//{{V2}}
FUNCTION_BLOCK FB32
TITLE=Get Homing Parameter
//*****************************************************************************
//* maxon motor ag
//* R&D
//* all rights reserved
//*****************************************************************************
//* Summary:  Read all homing parameters
//*
//* Remarks:
//*
//* Created under: STEP7 REV5.2+SP1
//*****************************************************************************
//* History:
//* 19.05.2004 | INA   first release
//*
//*
//*****************************************************************************
//


AUTHOR:INA
FAMILY:HomingMo
NAME:GetHoPa
VERSION:00.01


VAR_INPUT
       Read:BOOL //A rising edge start the command
       NodeID:BYTE //Adress of the maxon device
END_VAR

VAR_OUTPUT
       Done:BOOL //Data valid flag is TRUE if data were available
       Err:BOOL //Error flag is TRUE if an Error has occured, see ErrNo for more details
       ErrNo:DINT //Contains detailed error information
       HomingAcceleration:DWORD //Acceleration for Homing Profile
       SpeedSwitch:DWORD //Speed during search for switch
       SpeedIndex:DWORD //Speed during search for index signal
       HomeOffset:DINT //Home Offset after Homing
       CurrentThreshold:WORD //Current Threshold for Homing Method -3 and -4
       HomePosition:DINT //Home position value
END_VAR

VAR_IN_OUT
END_VAR

VAR
       xEdgeMerker:BOOL //Edge Merker
       xEdgeFlag:BOOL //Edge Flag
       xStep:INT
END_VAR

VAR_TEMP
END_VAR
BEGIN

NETWORK
TITLE= Activate the service function
//{{a}}
//

// SDO Read "Get Homing Parameter"

       U    #Read
       FP   #xEdgeFlag                   // recognize a positiv edge of the Read signal
       =    #xEdgeMerker                 // and set the xEdgeMerker for one cycle to true

       L    #xStep
       L    0
       ==I
       U    #xEdgeMerker
       SPB  nstp                         // iStep = 1 -> fnc1

       L    #xStep                       // jump list
       SPL  List
       SPA  rdef
       SPA  fnc1
       SPA  fncE
List  :SPA  rdef

rdef  :NOP  0
       R    #Done                        // reset Done
       R    #Err                         // reset Error
       L    0
       T    #xStep                       // iStep = 0
       SPA  end

fnc1  :NOP  0
       CALL FC1
         NodeID:=#NodeID
         Index:=DW#16#00006099
         SubIndex:=DW#16#00000002
         RET_VAL:=#Done
         Err:=#Err
         ErrNo:=#ErrNo

       L    DB219.DBD10
       T    #SpeedIndex

       L    1
       U    #Err
       SPB  fncE

       NOP  0
       CALL FC1
         NodeID:=#NodeID
         Index:=DW#16#0000609A
         SubIndex:=DW#16#00000000
         RET_VAL:=#Done
         Err:=#Err
         ErrNo:=#ErrNo

       L    DB219.DBD10
       T    #HomingAcceleration

       L    1
       U    #Err
       SPB  fncE

       NOP  0
       CALL FC1
         NodeID:=#NodeID
         Index:=DW#16#00006099
         SubIndex:=DW#16#00000001
         RET_VAL:=#Done
         Err:=#Err
         ErrNo:=#ErrNo

       L    DB219.DBD10
       T    #SpeedSwitch

       L    1
       U    #Err
       SPB  fncE

       NOP  0
       CALL FC1
         NodeID:=#NodeID
         Index:=DW#16#0000607C
         SubIndex:=DW#16#00000000
         RET_VAL:=#Done
         Err:=#Err
         ErrNo:=#ErrNo

       L    DB219.DBD10
       T    #HomeOffset

       L    1
       U    #Err
       SPB  fncE

       NOP  0
       CALL FC1
         NodeID:=#NodeID
         Index:=DW#16#00002080
         SubIndex:=DW#16#00000000
         RET_VAL:=#Done
         Err:=#Err
         ErrNo:=#ErrNo

       L    DB219.DBW10
       T    #CurrentThreshold

       L    1
       U    #Err
       SPB  fncE

       NOP  0
       CALL FC1
         NodeID:=#NodeID
         Index:=DW#16#00002081
         SubIndex:=DW#16#00000000
         RET_VAL:=#Done
         Err:=#Err
         ErrNo:=#ErrNo

       L    DB219.DBD10
       T    #HomePosition

fncE  :NOP  0
       L    0
       T    #xStep
       SPA  end

nstp  :NOP  0
       L    #xStep
       INC            1
       T    #xStep

end   :NOP  0
END_FUNCTION_BLOCK
